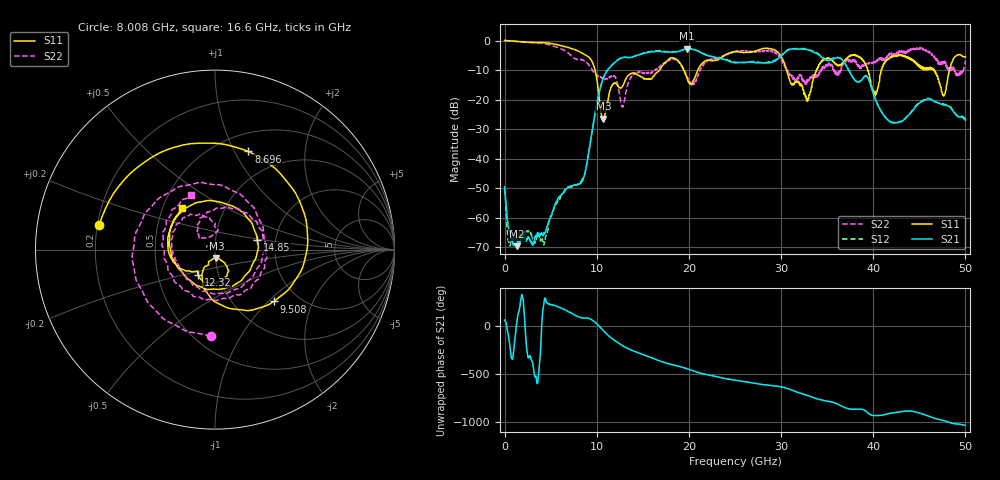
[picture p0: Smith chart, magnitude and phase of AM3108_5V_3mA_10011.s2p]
# Hz S DB R 50.0
!freq dBS11 angS11 dBS21 angS21 dBS12 angS12 dBS22 angS22
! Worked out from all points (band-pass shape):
!   1601 points, 10 MHz to 50 GHz, reference 50 ohm
!   highest |S21| = -2.76 dB at 19.82 GHz (marker M1); lowest = -69.7 dB at 1.353 GHz (marker M2)
!   |S21| within 3 dB of the highest: 13.72 GHz to 22.86 GHz (9.149 GHz wide, 50 % of centre); 29.82 GHz to 34.44 GHz (4.621 GHz wide, 14.4 % of centre)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
!   lowest |S11| = -26.5 dB at 10.73 GHz (marker M3), VSWR 1.10, Z = 50.6 - j4.71 ohm
!   |S11| at or under -10 dB: 9.818 GHz to 16.81 GHz (6.991 GHz wide, 52.5 % of centre); 30.61 GHz to 33.84 GHz (3.23 GHz wide, 10 % of centre); 46.63 GHz to 48.28 GHz (1.653 GHz wide, 3.48 % of centre)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
!   |S22| runs from -22.5 to 0.0 dB; largest |S21 - S12| = 0.022
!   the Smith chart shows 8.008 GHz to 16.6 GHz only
!   S11 on the Smith chart (normalised r, x): 8.008 GHz: 0.21, +0.10; 8.696 GHz: 0.69, +1.14; 9.508 GHz: 1.51, -1.08; 12.32 GHz: 0.80, -0.23; 14.85 GHz: 1.61, +0.18; 16.6 GHz: 0.63, +0.31
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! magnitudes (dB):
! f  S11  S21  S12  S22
! 10 MHz  0.0  -49.5  -50.5  0.0
! 509.9 MHz  -0.1  -64.2  -68.9  -0.2
! 1.353 GHz  -0.3  -69.7  -66.3  -0.4
! 4.228 GHz  -0.7  -65.9  -69.1  -1.1
! 8.008 GHz  -3.6  -48.7  -48.8  -6.4
! 8.352 GHz  -4.1  -48.1  -47.5  -6.4
! 8.696 GHz  -4.8  -45.4  -45.1  -6.9
! 9.508 GHz  -7.2  -30.6  -30.6  -9.9
! 10.73 GHz  -26.5  -12.6  -12.6  -12.8
! 12.32 GHz  -15.5  -6.5  -6.5  -15.3
! 14.85 GHz  -12.3  -4.6  -4.5  -10.6
! 16.6 GHz  -10.6  -3.7  -3.4  -9.5
! 16.69 GHz  -10.4  -3.6  -3.4  -9.5
! 19.82 GHz  -12.9  -2.8  -2.7  -12.6
! 25 GHz  -3.8  -7.5  -7.3  -3.8
! 29.25 GHz  -3.1  -7.1  -6.7  -3.9
! 33.35 GHz  -15.6  -3.7  -3.4  -12.7
! 38 GHz  -4.8  -13.4  -13.4  -6.6
! 40.22 GHz  -18.7  -19.8  -19.7  -7.6
! 41.69 GHz  -6.1  -27.2  -27.0  -5.2
! 47.66 GHz  -18.8  -21.9  -21.5  -7.7
! 50 GHz  -5.5  -27.0  -26.6  -6.9
